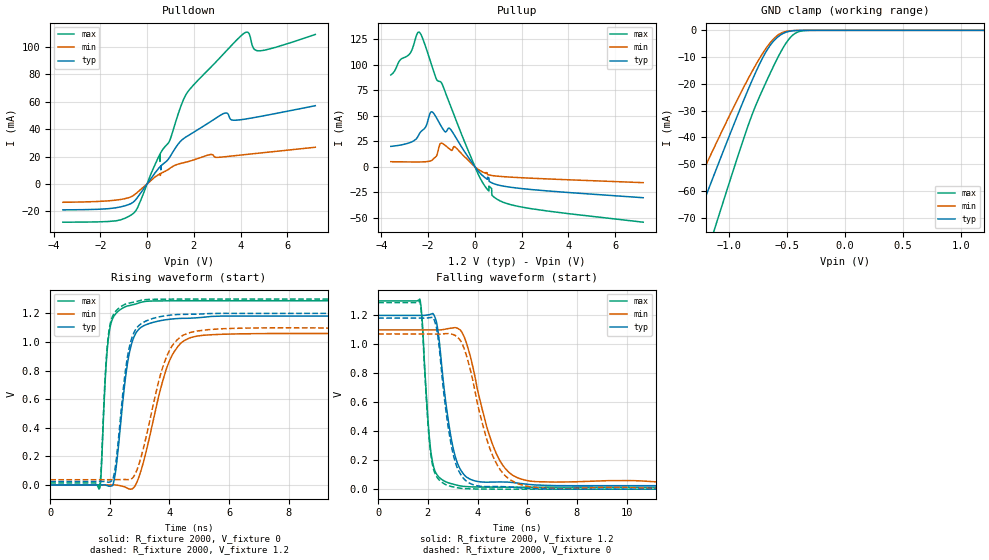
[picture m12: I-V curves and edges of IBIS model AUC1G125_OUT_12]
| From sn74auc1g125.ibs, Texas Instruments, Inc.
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[Model]   AUC1G125_OUT_12
Model_type  3-state
Enable   Active-Low
Vref =   0
Rref =   2000
Cref =   15p
Vmeas =   0.6
| variable   typ   min   max
C_comp   5.50pF   NA   NA
| C_pullup   10.79pF   3.24pF   21.90pF
| C_pulldown   11.71pF   5.76pF   22.04pF
| C_tri-state   9.31pF   5.49pF   18.87pF
[Temperature Range]   40   100   -40
| Ambient temperature   25   85   -40
[Voltage range]   1.2   1.1   1.3
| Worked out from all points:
|   slope of the pulldown table from 0 to 0.18 V, typ, clamps not added: 42.3 ohm
|   slope of the pullup table from 0 to 0.18 V, typ, clamps not added: 34.6 ohm
|   GND clamp passes 1 mA (typ) near -0.53 V on its own axis
|   rising waveform, R_fixture 2000, V_fixture 0: 20-80 % time 406ps typ, 786ps min, 210ps max; typ from 0 V to 1.18 V
|   falling waveform, R_fixture 2000, V_fixture 1.2: 20-80 % time 558ps typ, 993ps min, 299ps max; typ from 1.2 V to 0.024 V
|   rising waveform, R_fixture 2000, V_fixture 1.2: 20-80 % time 398ps typ, 771ps min, 207ps max; typ from 0.024 V to 1.2 V
|   falling waveform, R_fixture 2000, V_fixture 0: 20-80 % time 550ps typ, 994ps min, 295ps max; typ from 1.18 V to 0 V
[GND Clamp]
| AUC1G125_OUT_12
|   Voltage   I(typ)   I(min)   I(max)
-3.6V     -338.8mA   -286.3mA   -409.7mA
-1.445V   -89.45mA   -73.14mA   -117.7mA
-1.32V    -75.2mA    -61.33mA   -100.6mA
-1.28V    -70.67mA   -57.58mA   -95.15mA
-1.13V    -53.81mA   -43.72mA   -74.62mA
-1.095V   -49.91mA   -40.54mA   -69.84mA
-820mV    -20.45mA   -16.73mA   -33.53mA
-695mV    -8.981mA   -7.553mA   -20.59mA
-575mV    -2.299mA   -1.652mA   -9.733mA
-435mV    -119.5uA   -67.45uA   -1.256mA
-295mV    -1.95uA    -1.721uA   -13.96uA
1.2V      281.9pA    6.337nA    254pA
[Pulldown]
| AUC1G125_OUT_12
|   Voltage   I(typ)   I(min)   I(max)
-3.6V     -18.86mA   -13.33mA   -27.86mA
-535mV    -12.4mA    -7.815mA   -20.65mA
495mV     11.41mA    6.857mA    19.85mA
545mV     12.35mA    7.329mA    21.54mA
550mV     12.44mA    7.375mA    16.48mA
570mV     12.79mA    6.265mA    22.32mA
965mV     19.42mA    11.26mA    31.49mA
1.685V    34.52mA    16.01mA    65.78mA
3.32V     51.72mA    19.88mA    95.8mA
4.13V     47.2mA     21.35mA    109.8mA
4.785V    49.12mA    22.52mA    97.19mA
7.2V      57.15mA    26.83mA    109.1mA
[Pullup]
| AUC1G125_OUT_12
|   Voltage   I(typ)   I(min)   I(max)
-3.6V     20.02mA    4.99mA     89.94mA
-2.77V    23.81mA    4.762mA    111.3mA
-2.475V   28.39mA    4.727mA    130.3mA
-2.355V   33.26mA    4.746mA    131.3mA
-1.82V    53.68mA    6.71mA     97.32mA
-1.635V   47.58mA    11.11mA    85.27mA
-1.43V    39.24mA    23.25mA    82.18mA
-1.05V    36.9mA     16.86mA    60mA
-860mV    30.31mA    19.57mA    48.76mA
155mV     -4.519mA   -2.712mA   -8.028mA
970mV     -17.73mA   -9.185mA   -32.13mA
7.2V      -30.3mA    -15.54mA   -54.28mA
[Ramp]
| AUC1G125_OUT_12
| variable   typ   min   max
dV/dt_r   0.71/4.12E-10   0.66/8.31E-10   0.79/2.15E-10
dV/dt_f   0.71/5.64E-10   0.65/1.03E-09   0.78/3.03E-10
R_load = 2000
[Rising Waveform]
| AUC1G125_OUT_12
R_fixture =   2000
C_fixture =   0
L_fixture =   0
V_fixture =   0
V_fixture_min = 0
V_fixture_max = 0
|   Time   V(typ)   V(min)   V(max)
0s        5.968nV    25.09nV    694.9pV
1.665ns   127.3uV    -16.51uV   -18.37mV
1.895ns   -3.172mV   103.3uV    899.4mV
2.095ns   -3.694mV   620.4uV    1.164V
2.215ns   129.1mV    -352.2uV   1.202V
2.64ns    907.5mV    -27.05mV   1.254V
3.125ns   1.112V     158.3mV    1.281V
4.005ns   1.159V     869.8mV    1.288V
4.935ns   1.169V     1.042V     1.288V
29.99ns   1.181V     1.072V     1.288V
[Falling Waveform]
| AUC1G125_OUT_12
R_fixture =   2000
C_fixture =   0
L_fixture =   0
V_fixture =   1.2
V_fixture_min = 1.1
V_fixture_max = 1.3
|   Time   V(typ)   V(min)   V(max)
0s        1.2V       1.1V       1.3V
1.68ns    1.2V       1.1V       1.312V
2.045ns   1.205V     1.1V       387.3mV
2.245ns   1.203V     1.1V       146.6mV
2.855ns   438.3mV    1.11V      42.2mV
3.145ns   201.6mV    1.114V     28.46mV
3.565ns   82.28mV    1.003V     17.51mV
4.755ns   49.36mV    245.8mV    13.89mV
5.925ns   35.41mV    61.64mV    13.8mV
29.99ns   23.98mV    36.64mV    13.86mV
[Rising Waveform]
| AUC1G125_OUT_12
R_fixture =   2000
C_fixture =   0
L_fixture =   0
V_fixture =   1.2
V_fixture_min = 1.1
V_fixture_max = 1.3
|   Time   V(typ)   V(min)   V(max)
0s        23.98mV    36.64mV    13.86mV
1.655ns   24.06mV    36.64mV    -2.318mV
1.705ns   24.15mV    36.64mV    101mV
1.895ns   22.02mV    36.71mV    927.2mV
2.095ns   34.98mV    36.96mV    1.181V
2.615ns   923.7mV    37.5mV     1.27V
3.065ns   1.13V      208.5mV    1.292V
3.94ns    1.185V     914.3mV    1.299V
4.92ns    1.194V     1.076V     1.3V
29.99ns   1.2V       1.1V       1.3V
[Falling Waveform]
| AUC1G125_OUT_12
R_fixture =   2000
C_fixture =   0
L_fixture =   0
V_fixture =   0
V_fixture_min = 0
V_fixture_max = 0
|   Time   V(typ)   V(min)   V(max)
0s        1.181V     1.072V     1.288V
1.68ns    1.181V     1.072V     1.299V
2.005ns   1.183V     1.071V     449.9mV
2.145ns   1.186V     1.071V     207.4mV
2.38ns    1.082V     1.071V     79.42mV
2.93ns    314.5mV    1.072V     18.99mV
3.485ns   65.06mV    959.4mV    3.811mV
4.69ns    18.31mV    200.9mV    94.93uV
5.89ns    6.651mV    23.64mV    -57.68uV
29.99ns   3.948uV    -1.05uV    82.98nV
